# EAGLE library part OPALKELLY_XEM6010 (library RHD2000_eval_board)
Opal Kelly XEM6010 USB/FPGA module
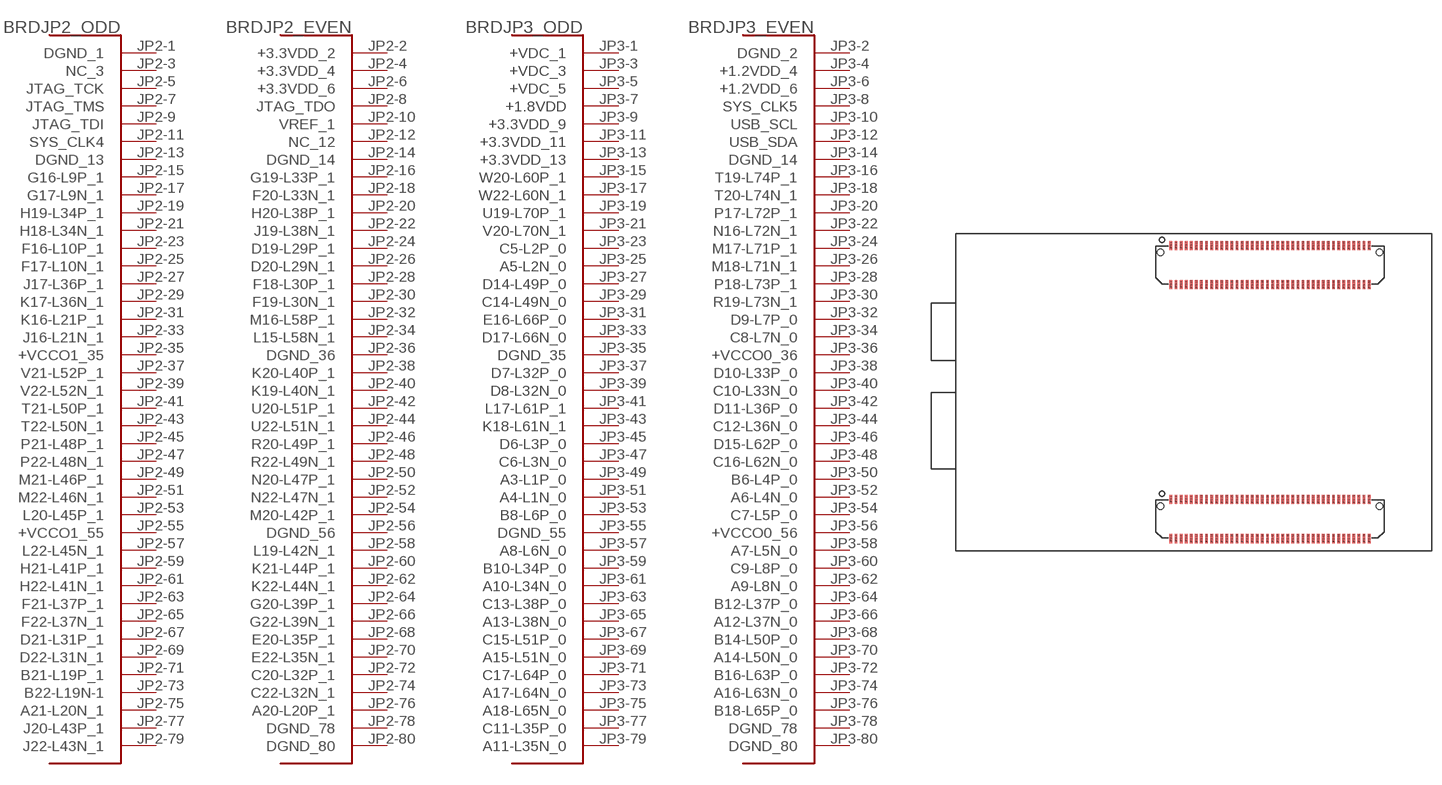
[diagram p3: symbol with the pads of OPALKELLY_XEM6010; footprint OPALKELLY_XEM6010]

Designator prefix BRD; gates JP2_ODD=XEM6010_JP2_ODD JP2_EVEN=XEM6010_JP2_EVEN JP3_ODD=XEM6010_JP3_ODD JP3_EVEN=XEM6010_JP3_EVEN

## OPALKELLY_XEM6010  [OPALKELLY_XEM6010]
JP2-1  JP2_ODD:DGND_1  pwr
JP2-2  JP2_EVEN:+3.3VDD_2  pwr
JP2-3  JP2_ODD:NC_3  nc
JP2-4  JP2_EVEN:+3.3VDD_4  pwr
JP2-5  JP2_ODD:JTAG_TCK
JP2-6  JP2_EVEN:+3.3VDD_6  pwr
JP2-7  JP2_ODD:JTAG_TMS
JP2-8  JP2_EVEN:JTAG_TDO
JP2-9  JP2_ODD:JTAG_TDI
JP2-10  JP2_EVEN:VREF_1  in
JP2-11  JP2_ODD:SYS_CLK4  out
JP2-12  JP2_EVEN:NC_12  nc
JP2-13  JP2_ODD:DGND_13  pwr
JP2-14  JP2_EVEN:DGND_14  pwr
JP2-15  JP2_ODD:G16-L9P_1
JP2-16  JP2_EVEN:G19-L33P_1
JP2-17  JP2_ODD:G17-L9N_1
JP2-18  JP2_EVEN:F20-L33N_1
JP2-19  JP2_ODD:H19-L34P_1
JP2-20  JP2_EVEN:H20-L38P_1
JP2-21  JP2_ODD:H18-L34N_1
JP2-22  JP2_EVEN:J19-L38N_1
JP2-23  JP2_ODD:F16-L10P_1
JP2-24  JP2_EVEN:D19-L29P_1
JP2-25  JP2_ODD:F17-L10N_1
JP2-26  JP2_EVEN:D20-L29N_1
JP2-27  JP2_ODD:J17-L36P_1
JP2-28  JP2_EVEN:F18-L30P_1
JP2-29  JP2_ODD:K17-L36N_1
JP2-30  JP2_EVEN:F19-L30N_1
JP2-31  JP2_ODD:K16-L21P_1
JP2-32  JP2_EVEN:M16-L58P_1
JP2-33  JP2_ODD:J16-L21N_1
JP2-34  JP2_EVEN:L15-L58N_1
JP2-35  JP2_ODD:+VCCO1_35  pwr
JP2-36  JP2_EVEN:DGND_36  pwr
JP2-37  JP2_ODD:V21-L52P_1
JP2-38  JP2_EVEN:K20-L40P_1
JP2-39  JP2_ODD:V22-L52N_1
JP2-40  JP2_EVEN:K19-L40N_1
JP2-41  JP2_ODD:T21-L50P_1
JP2-42  JP2_EVEN:U20-L51P_1
JP2-43  JP2_ODD:T22-L50N_1
JP2-44  JP2_EVEN:U22-L51N_1
JP2-45  JP2_ODD:P21-L48P_1
JP2-46  JP2_EVEN:R20-L49P_1
JP2-47  JP2_ODD:P22-L48N_1
JP2-48  JP2_EVEN:R22-L49N_1
JP2-49  JP2_ODD:M21-L46P_1
JP2-50  JP2_EVEN:N20-L47P_1
JP2-51  JP2_ODD:M22-L46N_1
JP2-52  JP2_EVEN:N22-L47N_1
JP2-53  JP2_ODD:L20-L45P_1
JP2-54  JP2_EVEN:M20-L42P_1
JP2-55  JP2_ODD:+VCCO1_55  pwr
JP2-56  JP2_EVEN:DGND_56  pwr
JP2-57  JP2_ODD:L22-L45N_1
JP2-58  JP2_EVEN:L19-L42N_1
JP2-59  JP2_ODD:H21-L41P_1
JP2-60  JP2_EVEN:K21-L44P_1
JP2-61  JP2_ODD:H22-L41N_1
JP2-62  JP2_EVEN:K22-L44N_1
JP2-63  JP2_ODD:F21-L37P_1
JP2-64  JP2_EVEN:G20-L39P_1
JP2-65  JP2_ODD:F22-L37N_1
JP2-66  JP2_EVEN:G22-L39N_1
JP2-67  JP2_ODD:D21-L31P_1
JP2-68  JP2_EVEN:E20-L35P_1
JP2-69  JP2_ODD:D22-L31N_1
JP2-70  JP2_EVEN:E22-L35N_1
JP2-71  JP2_ODD:B21-L19P_1
JP2-72  JP2_EVEN:C20-L32P_1
JP2-73  JP2_ODD:B22-L19N-1
JP2-74  JP2_EVEN:C22-L32N_1
JP2-75  JP2_ODD:A21-L20N_1
JP2-76  JP2_EVEN:A20-L20P_1
JP2-77  JP2_ODD:J20-L43P_1
JP2-78  JP2_EVEN:DGND_78  pwr
JP2-79  JP2_ODD:J22-L43N_1
JP2-80  JP2_EVEN:DGND_80  pwr
JP3-1  JP3_ODD:+VDC_1  pwr
JP3-2  JP3_EVEN:DGND_2  pwr
JP3-3  JP3_ODD:+VDC_3  pwr
JP3-4  JP3_EVEN:+1.2VDD_4  pwr
JP3-5  JP3_ODD:+VDC_5  pwr
JP3-6  JP3_EVEN:+1.2VDD_6  pwr
JP3-7  JP3_ODD:+1.8VDD  pwr
JP3-8  JP3_EVEN:SYS_CLK5  out
JP3-9  JP3_ODD:+3.3VDD_9  pwr
JP3-10  JP3_EVEN:USB_SCL
JP3-11  JP3_ODD:+3.3VDD_11  pwr
JP3-12  JP3_EVEN:USB_SDA
JP3-13  JP3_ODD:+3.3VDD_13  pwr
JP3-14  JP3_EVEN:DGND_14  pwr
JP3-15  JP3_ODD:W20-L60P_1
JP3-16  JP3_EVEN:T19-L74P_1
JP3-17  JP3_ODD:W22-L60N_1
JP3-18  JP3_EVEN:T20-L74N_1
JP3-19  JP3_ODD:U19-L70P_1
JP3-20  JP3_EVEN:P17-L72P_1
JP3-21  JP3_ODD:V20-L70N_1
JP3-22  JP3_EVEN:N16-L72N_1
JP3-23  JP3_ODD:C5-L2P_0
JP3-24  JP3_EVEN:M17-L71P_1
JP3-25  JP3_ODD:A5-L2N_0
JP3-26  JP3_EVEN:M18-L71N_1
JP3-27  JP3_ODD:D14-L49P_0
JP3-28  JP3_EVEN:P18-L73P_1
JP3-29  JP3_ODD:C14-L49N_0
JP3-30  JP3_EVEN:R19-L73N_1
JP3-31  JP3_ODD:E16-L66P_0
JP3-32  JP3_EVEN:D9-L7P_0
JP3-33  JP3_ODD:D17-L66N_0
JP3-34  JP3_EVEN:C8-L7N_0
JP3-35  JP3_ODD:DGND_35  pwr
JP3-36  JP3_EVEN:+VCCO0_36  pwr
JP3-37  JP3_ODD:D7-L32P_0
JP3-38  JP3_EVEN:D10-L33P_0
JP3-39  JP3_ODD:D8-L32N_0
JP3-40  JP3_EVEN:C10-L33N_0
JP3-41  JP3_ODD:L17-L61P_1
JP3-42  JP3_EVEN:D11-L36P_0
JP3-43  JP3_ODD:K18-L61N_1
JP3-44  JP3_EVEN:C12-L36N_0
JP3-45  JP3_ODD:D6-L3P_0
JP3-46  JP3_EVEN:D15-L62P_0
JP3-47  JP3_ODD:C6-L3N_0
JP3-48  JP3_EVEN:C16-L62N_0
JP3-49  JP3_ODD:A3-L1P_0
JP3-50  JP3_EVEN:B6-L4P_0
JP3-51  JP3_ODD:A4-L1N_0
JP3-52  JP3_EVEN:A6-L4N_0
JP3-53  JP3_ODD:B8-L6P_0
JP3-54  JP3_EVEN:C7-L5P_0
JP3-55  JP3_ODD:DGND_55  pwr
JP3-56  JP3_EVEN:+VCCO0_56  pwr
JP3-57  JP3_ODD:A8-L6N_0
JP3-58  JP3_EVEN:A7-L5N_0
JP3-59  JP3_ODD:B10-L34P_0
JP3-60  JP3_EVEN:C9-L8P_0
JP3-61  JP3_ODD:A10-L34N_0
JP3-62  JP3_EVEN:A9-L8N_0
JP3-63  JP3_ODD:C13-L38P_0
JP3-64  JP3_EVEN:B12-L37P_0
JP3-65  JP3_ODD:A13-L38N_0
JP3-66  JP3_EVEN:A12-L37N_0
JP3-67  JP3_ODD:C15-L51P_0
JP3-68  JP3_EVEN:B14-L50P_0
JP3-69  JP3_ODD:A15-L51N_0
JP3-70  JP3_EVEN:A14-L50N_0
JP3-71  JP3_ODD:C17-L64P_0
JP3-72  JP3_EVEN:B16-L63P_0
JP3-73  JP3_ODD:A17-L64N_0
JP3-74  JP3_EVEN:A16-L63N_0
JP3-75  JP3_ODD:A18-L65N_0
JP3-76  JP3_EVEN:B18-L65P_0
JP3-77  JP3_ODD:C11-L35P_0
JP3-78  JP3_EVEN:DGND_78  pwr
JP3-79  JP3_ODD:A11-L35N_0
JP3-80  JP3_EVEN:DGND_80  pwr

## Footprint OPALKELLY_XEM6010 (pad centres in mm)
smd 0.457 x 1.448: JP2-1 33.9,8.086; JP2-2 33.9,1.914; JP2-3 34.7,8.086; JP2-4 34.7,1.914; JP2-5 35.5,8.086; JP2-6 35.5,1.914; JP2-7 36.3,8.086; JP2-8 36.3,1.914; JP2-9 37.1,8.086; JP2-10 37.1,1.914; JP2-11 37.9,8.086; JP2-12 37.9,1.914; JP2-13 38.7,8.086; JP2-14 38.7,1.914; JP2-15 39.5,8.086; JP2-16 39.5,1.914; JP2-17 40.3,8.086; JP2-18 40.3,1.914; JP2-19 41.1,8.086; JP2-20 41.1,1.914; JP2-21 41.9,8.086; JP2-22 41.9,1.914; JP2-23 42.7,8.086; JP2-24 42.7,1.914; JP2-25 43.5,8.086; JP2-26 43.5,1.914; JP2-27 44.3,8.086; JP2-28 44.3,1.914; JP2-29 45.1,8.086; JP2-30 45.1,1.914; JP2-31 45.9,8.086; JP2-32 45.9,1.914; JP2-33 46.7,8.086; JP2-34 46.7,1.914; JP2-35 47.5,8.086; JP2-36 47.5,1.914; JP2-37 48.3,8.086; JP2-38 48.3,1.914; JP2-39 49.1,8.086; JP2-40 49.1,1.914; JP2-41 49.9,8.086; JP2-42 49.9,1.914; JP2-43 50.7,8.086; JP2-44 50.7,1.914; JP2-45 51.5,8.086; JP2-46 51.5,1.914; JP2-47 52.3,8.086; JP2-48 52.3,1.914; JP2-49 53.1,8.086; JP2-50 53.1,1.914; JP2-51 53.9,8.086; JP2-52 53.9,1.914; JP2-53 54.7,8.086; JP2-54 54.7,1.914; JP2-55 55.5,8.086; JP2-56 55.5,1.914; JP2-57 56.3,8.086; JP2-58 56.3,1.914; JP2-59 57.1,8.086; JP2-60 57.1,1.914; JP2-61 57.9,8.086; JP2-62 57.9,1.914; JP2-63 58.7,8.086; JP2-64 58.7,1.914; JP2-65 59.5,8.086; JP2-66 59.5,1.914; JP2-67 60.3,8.086; JP2-68 60.3,1.914; JP2-69 61.1,8.086; JP2-70 61.1,1.914; JP2-71 61.9,8.086; JP2-72 61.9,1.914; JP2-73 62.7,8.086; JP2-74 62.7,1.914; JP2-75 63.5,8.086; JP2-76 63.5,1.914; JP2-77 64.3,8.086; JP2-78 64.3,1.914; JP2-79 65.1,8.086; JP2-80 65.1,1.914; JP3-1 33.9,48.086; JP3-2 33.9,41.914; JP3-3 34.7,48.086; JP3-4 34.7,41.914; JP3-5 35.5,48.086; JP3-6 35.5,41.914; JP3-7 36.3,48.086; JP3-8 36.3,41.914; JP3-9 37.1,48.086; JP3-10 37.1,41.914; JP3-11 37.9,48.086; JP3-12 37.9,41.914; JP3-13 38.7,48.086; JP3-14 38.7,41.914; JP3-15 39.5,48.086; JP3-16 39.5,41.914; JP3-17 40.3,48.086; JP3-18 40.3,41.914; JP3-19 41.1,48.086; JP3-20 41.1,41.914; JP3-21 41.9,48.086; JP3-22 41.9,41.914; JP3-23 42.7,48.086; JP3-24 42.7,41.914; JP3-25 43.5,48.086; JP3-26 43.5,41.914; JP3-27 44.3,48.086; JP3-28 44.3,41.914; JP3-29 45.1,48.086; JP3-30 45.1,41.914; JP3-31 45.9,48.086; JP3-32 45.9,41.914; JP3-33 46.7,48.086; JP3-34 46.7,41.914; JP3-35 47.5,48.086; JP3-36 47.5,41.914; JP3-37 48.3,48.086; JP3-38 48.3,41.914; JP3-39 49.1,48.086; JP3-40 49.1,41.914; JP3-41 49.9,48.086; JP3-42 49.9,41.914; JP3-43 50.7,48.086; JP3-44 50.7,41.914; JP3-45 51.5,48.086; JP3-46 51.5,41.914; JP3-47 52.3,48.086; JP3-48 52.3,41.914; JP3-49 53.1,48.086; JP3-50 53.1,41.914; JP3-51 53.9,48.086; JP3-52 53.9,41.914; JP3-53 54.7,48.086; JP3-54 54.7,41.914; JP3-55 55.5,48.086; JP3-56 55.5,41.914; JP3-57 56.3,48.086; JP3-58 56.3,41.914; JP3-59 57.1,48.086; JP3-60 57.1,41.914; JP3-61 57.9,48.086; JP3-62 57.9,41.914; JP3-63 58.7,48.086; JP3-64 58.7,41.914; JP3-65 59.5,48.086; JP3-66 59.5,41.914; JP3-67 60.3,48.086; JP3-68 60.3,41.914; JP3-69 61.1,48.086; JP3-70 61.1,41.914; JP3-71 61.9,48.086; JP3-72 61.9,41.914; JP3-73 62.7,48.086; JP3-74 62.7,41.914; JP3-75 63.5,48.086; JP3-76 63.5,41.914; JP3-77 64.3,48.086; JP3-78 64.3,41.914; JP3-79 65.1,48.086; JP3-80 65.1,41.914
hole 1.016 at 32.261,47.032
hole 1.016 at 66.739,47.032
hole 1.016 at 32.261,7.032
hole 1.016 at 66.739,7.032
